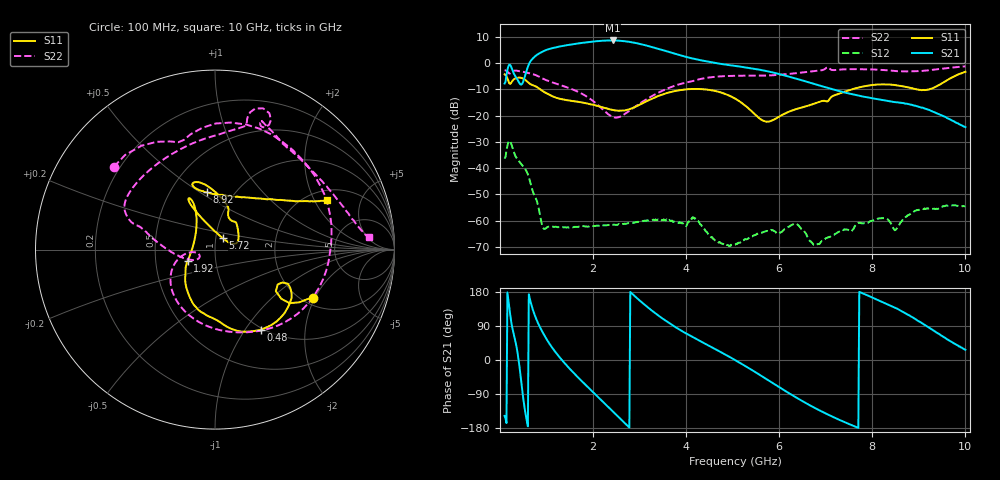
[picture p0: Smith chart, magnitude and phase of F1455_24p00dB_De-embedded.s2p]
! Integrated Device Technology
! Corporate Headquarters
! 6024 Silver Creek Valley Road
! San Jose, CA 95138  USA
! Phone:  1-408-284-8200
! Toll Free:  1-800-223-1366
! Webpage:  http://www.idt.com/
! Timing and RF Division
! 515 Groton Road, Suite 102
! Westford, MA 01886-6024
! Device:  F1455
! Description: 6-bit 0.5 dB Transmit Variable Gain Amplifier
! Frequency:  1400.0 -  2300.00 MHz
! Package:  6x6 mm Thin QFN Plastic Package: 28 pin
! State:  48
! Atten State:  24.0 dB
! Voltage:  +5.00 Volts
! Current:  217.642 mA
! Data:  The device was measured on a the F1455 evaluation board which has
!  individual transmission lines to the RF pins.  Data was collected
!  using a calibrated network analyzer.  The evaluation board was
!  de-embedded using a TRL calibration technique.
!  The reference plane is the edge of the package pin.
!  Pin  1 = CSb
!  Pin  2 = DATA
!  Pin  3 = CLK
!  Pin  4 = RSET
!  Pin  5 = GND
!  Pin  6 = RFIN  = Port 1
!  Pin  7 = GND
!  Pin  8 = NC
!  Pin  9 = NC
!  Pin 10 = NC
!  Pin 11 = NC
!  Pin 12 = NC
!  Pin 13 = NC
!  Pin 14 = /STBY
!  Pin 15 = GND
!  Pin 16 = RFOUT  = Port 2
!  Pin 17 = GND
!  Pin 18 = NC
!  Pin 19 = NC
!  Pin 20 = NC
!  Pin 21 = GND
!  Pin 22 = NC
!  Pin 23 = GND
!  Pin 24 = NC
!  Pin 25 = NC
!  Pin 26 = NC
!  Pin 27 = GND
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# GHz S dB R 50
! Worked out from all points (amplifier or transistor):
!   496 points, 100 MHz to 10 GHz, reference 50 ohm
!   highest |S21| = 8.6 dB at 2.42 GHz (marker M1)
!   |S21| within 3 dB of that: 1.111 GHz to 3.366 GHz (2.255 GHz wide, 101 % of centre)
!   unconditionally stable (mu >= 1): start of sweep to end of sweep
!   at 1.74 GHz: K = 240.21, MAG = 8.1 dB, |S12| = -62.2 dB
!   at 5.06 GHz: K = 1037.33, MAG = 0.8 dB, |S12| = -69.0 dB
!   at 10 GHz: K = 599.54, MAG = -15.8 dB, |S12| = -54.5 dB
!   S11 on the Smith chart (normalised r, x): 100 MHz: 2.27, -1.94; 480 MHz: 0.97, -1.18; 1.92 GHz: 0.73, -0.10; 5.72 GHz: 1.08, +0.14; 8.92 GHz: 0.75, +0.53; 10 GHz: 2.45, +2.53
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0.1  -4.30 -26.1  -7.80 -147.4  -36.37 47.5  -2.75 140.7
0.18  -6.74 -36.6  -1.31 160.3  -30.18 -6.8  -3.71 112.5
0.26  -6.96 -25.1  -2.33 88.2  -31.70 -77.1  -3.32 96.0
0.38  -5.60 -42.4  -6.43 17.4  -36.72 -118.2  -3.00 58.0
0.48  -5.78 -60.4  -7.86 -81.0  -38.90 -149.7  -3.27 31.5
0.66  -8.07 -88.1  0.75 152.7  -46.04 141.8  -4.01 -10.8
0.8  -9.21 -106.0  3.16 102.4  -52.89 113.5  -4.85 -42.0
0.96  -11.12 -123.5  4.71 63.8  -63.08 128.6  -6.26 -71.4
1.34  -13.79 -143.5  6.47 -1.4  -62.43 107.6  -8.63 -121.2
1.76  -14.99 -153.6  7.64 -56.0  -61.99 77.5  -11.68 -156.0
1.92  -15.59 -156.9  8.00 -75.3  -62.18 69.9  -13.43 -165.3
2.16  -16.66 -165.2  8.42 -104.1  -61.75 60.2  -16.84 -173.6
2.42  -17.84 179.5  8.58 -135.4  -61.60 52.7  -20.50 -165.1
2.82  -17.32 142.9  7.93 177.1  -60.83 43.1  -17.69 -154.0
3.4  -12.54 117.0  5.40 117.7  -59.47 23.7  -11.33 178.9
4.08  -9.92 116.3  1.96 64.6  -59.51 9.8  -7.12 162.9
5.06  -13.62 114.6  -1.13 -0.7  -69.04 17.1  -4.85 147.9
5.72  -22.32 55.6  -3.04 -50.0  -63.96 20.4  -4.76 120.9
6.7  -15.80 37.2  -7.69 -122.3  -68.29 -138.8  -3.19 78.4
8.36  -8.18 108.5  -14.53 144.9  -60.00 74.0  -2.82 62.4
8.92  -9.83 98.0  -16.22 108.5  -56.20 97.3  -3.15 39.9
10  -3.33 23.9  -24.39 26.9  -54.47 26.2  -1.28 4.6
